// TwinCAT 3 PLC project UPS_usb_test
// ProgramVersion: 3.1.4023.0
// libraries:
//   Tc2_IoFunctions, * (Beckhoff Automation GmbH)
//   Tc2_Standard, * (Beckhoff Automation GmbH)
//   Tc2_System, * (Beckhoff Automation GmbH)
//   Tc3_Module, * (Beckhoff Automation GmbH)
// project tree:
//   DUTs/ dataDUT.TcDUT
//   / PlcTask.TcTTO
//   POUs/ MAIN.TcPOU
// real-time tasks:
//   TASK PlcTask: cycle T#10ms, priority 20, ADS port 350

CONFIGURATION UPS_usb_test
    RESOURCE PLC ON TwinCAT3
        TASK PlcTask(INTERVAL := T#10ms, PRIORITY := 20);
        PROGRAM MAIN WITH PlcTask : MAIN;
    END_RESOURCE
END_CONFIGURATION

// ---- DUTs/dataDUT.TcDUT
TYPE dataDUT :
STRUCT
	name:WSTRING;
	old:INT;
	sex:WSTRING;
	height:WSTRING;
	weight:WSTRING;
END_STRUCT
END_TYPE

// ---- POUs/MAIN.TcPOU
PROGRAM MAIN
VAR
	FB_GetUPSStatus: FB_GetUPSStatus;	
	dataloaded: BOOL;								//UPS数据文件读取状态（True为读取成功，False为读取失败）
	OldData: BOOL;									//UPS备份数据文件读取状态
	PersistentDataStatus: EPlcPersistentStatus;		//Persistent数据读取（恢复）状态
END_VAR
VAR PERSISTENT
	//设定的Persistent数据变量
	Int_persistent: INT;
	Float_persistent: LREAL;
	struct_persistent: dataDUT;
	Array_persistent: ARRAY[0..1048575] OF BYTE;
END_VAR

FB_GetUPSStatus(
	sNetId:= , 					//默认为本机Netid
	nPort:= , 					//ADS端口号，若不填写功能块会自动获取，默认0
	bEnable:= , 				//高电平有效，置True后循环读取UPS状态
	bValid=> , 					//当bValid为True时，stStatus的值有效
	bError=> , 
	nErrId=> , 
	stStatus=> );				//包含UPS信息的结构体
	

dataloaded:=_Appinfo.BootDataLoaded;
OldData:=_Appinfo.OldBootData;
PersistentDataStatus:=_Appinfo.PersistentStatus;

END_PROGRAM
